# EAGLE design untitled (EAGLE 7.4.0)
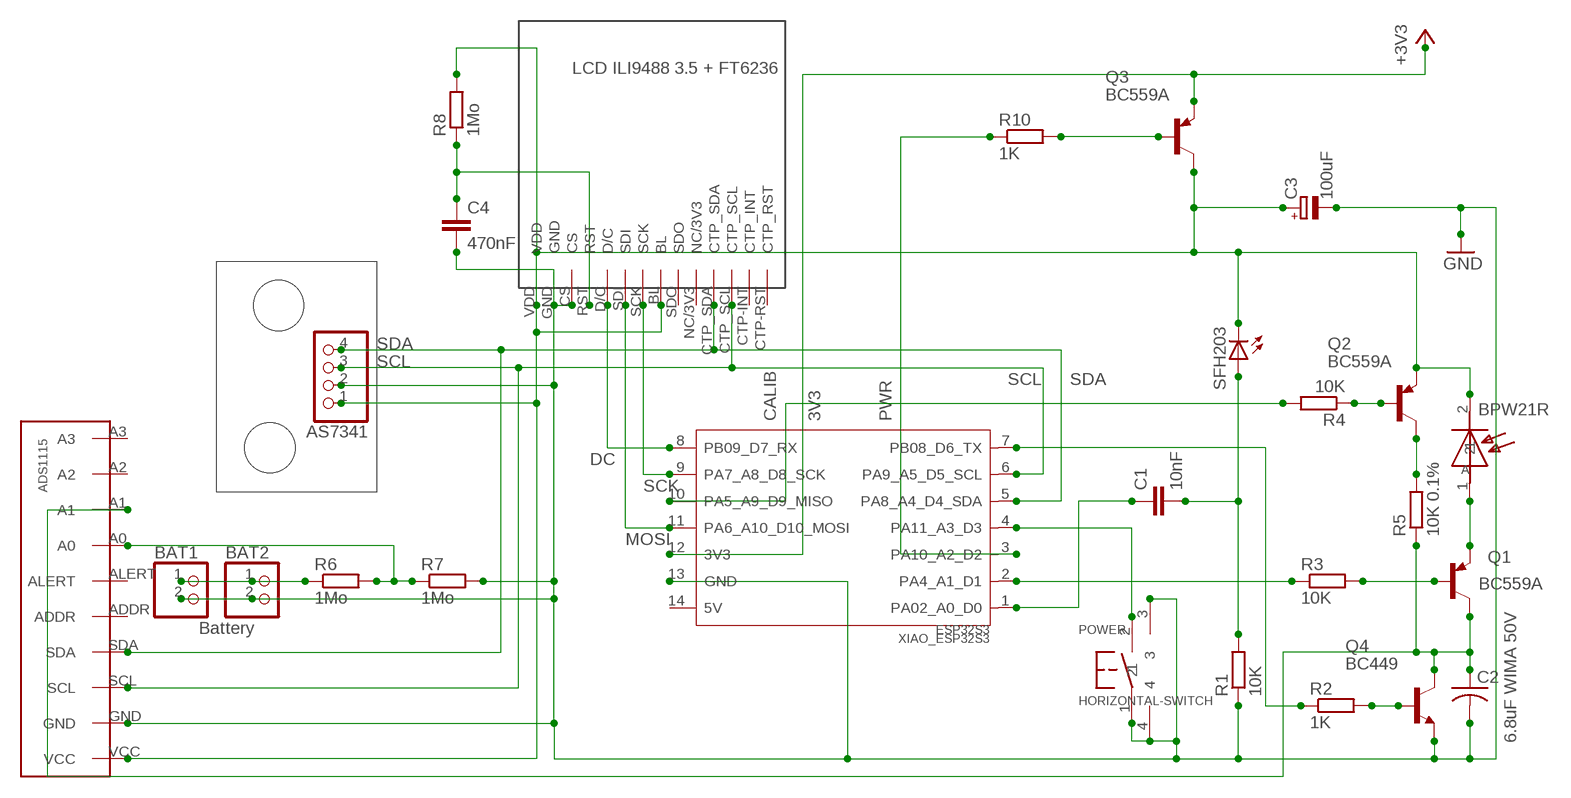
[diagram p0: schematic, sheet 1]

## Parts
ADS1115  HW-ADS1115  [HW-ADS1115]
AS7341  PINHD-1X4  [1X04]
BAT1  PINHD-1X2  [1X02]
BAT2  PINHD-1X2  [1X02]
BPW21R  BPW21  [BPW21]
C1  10nF  C-EU050-025X075  [C050-025X075]
C2  6.8uF WIMA 50V  C-US050-050X075  [C050-050X075]
C3  100uF  CPOL-EUE2.5-6  [E2,5-6]
C4  470nF  C-EU050-025X075  [C050-025X075]
LCD  LCD  IPS-ILI9488-3.5-480-320-FT6236  [IPS-ILI9488-3.5-480-320-FT6236]
POWER  HORIZONTAL-SWITCH  [HORIZONTAL-SWITCH]
Q1  BC559A  [TO92-EBC]
Q2  BC559A  [TO92-EBC]
Q3  BC559A  [TO92-EBC]
Q4  BC449  [TO92-EBC]
R1  10K  R-EU_0207/2V  [0207/2V]
R2  1K  R-EU_0207/2V  [0207/2V]
R3  10K  R-EU_0207/2V  [0207/2V]
R4  10K  R-EU_0207/2V  [0207/2V]
R5  10K 0.1%  R-EU_0207/2V  [0207/2V]
R6  1Mo  R-EU_0207/2V  [0207/2V]
R7  1Mo  R-EU_0207/2V  [0207/2V]
R8  1Mo  R-EU_0207/2V  [0207/2V]
R10  1K  R-EU_0207/2V  [0207/2V]
SFH203  SFH203  [SFH203]
XIAO_ESP32S3  ESP32S3  [MOUDLE14P-2.54-21X17.8MM]

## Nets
+3V3: Q3.E XIAO_ESP32S3.12(3V3)
GND: ADS1115.GND AS7341.2 BAT1.2 BAT2.2 C2.2 C3.- C4.2 LCD.CS LCD.GND POWER.1 POWER.3 POWER.4 Q4.E R1.1 R7.2 XIAO_ESP32S3.13(GND)
N$1: C4.1 LCD.RST R8.1
N$2: C1.1 XIAO_ESP32S3.1(PA02_A0_D0)
N$3: ADS1115.SCL AS7341.3 LCD.CTP_SCL XIAO_ESP32S3.6(PA9_A5_D5_SCL)
N$4: ADS1115.SDA AS7341.4 LCD.CTP_SDA XIAO_ESP32S3.5(PA8_A4_D4_SDA)
N$5: ADS1115.A0 R6.2 R7.1
N$6: LCD.SCK XIAO_ESP32S3.9(PA7_A8_D8_SCK)
N$7: LCD.SDI XIAO_ESP32S3.11(PA6_A10_D10_MOSI)
N$8: LCD.D/C XIAO_ESP32S3.8(PB09_D7_RX)
N$11: R10.1 XIAO_ESP32S3.3(PA10_A2_D2)
N$13: C1.2 R1.2 SFH203.A
N$14: BAT1.1 BAT2.1 R6.1
N$15: Q3.B R10.2
N$17: POWER.2 XIAO_ESP32S3.4(PA11_A3_D3)
N$18: ADS1115.VCC AS7341.1 BPW21R.2 C3.+ LCD.BL LCD.VDD Q2.E Q3.C R8.2 SFH203.K(C)
N$22: Q2.B R4.1
N$23: Q1.B R3.2
N$24: Q4.B R2.2
N$25: ADS1115.A1 C2.1 Q1.C Q4.C R5.1
N$26: Q2.C R5.2
N$27: BPW21R.1 Q1.E
N$29: R4.2 XIAO_ESP32S3.10(PA5_A9_D9_MISO)
N$30: R3.1 XIAO_ESP32S3.2(PA4_A1_D1)
N$31: R2.1 XIAO_ESP32S3.7(PB08_D6_TX)
Unconnected: ADS1115.A2 ADS1115.A3 ADS1115.ADDR ADS1115.ALERT LCD.CTP-INT(CTP_INT) LCD.CTP-RST(CTP_RST) LCD.NC/3V3 LCD.SDO XIAO_ESP32S3.14(5V)

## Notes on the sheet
- LCD ILI9488 3.5 + FT6236
- SDA
- SCL
- SCL | SDA
- CALIB | 3V3 | PWR
- DC
- SCK
- MOSI
- Battery

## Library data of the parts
ADS1115 = perso:HW-ADS1115
AS7341 = pinhead:PINHD-1X4: PIN HEADER
BAT1 BAT2 = pinhead:PINHD-1X2: PIN HEADER
BPW21R = perso:BPW21
C1 C4 = resistor:C-EU: CAPACITOR, European symbol
C2 = resistor:C-US: CAPACITOR, American symbol
C3 = resistor:CPOL-EU: POLARIZED CAPACITOR, European symbol
LCD = perso:IPS-ILI9488-3.5-480-320-FT6236
POWER = perso:HORIZONTAL-SWITCH
Q1-Q3 = transistor-pnp:BC559*: PNP Transistror
Q4 = transistor-npn:BC449*: NPN Transistor
R1-R8 R10 = resistor:R-EU_: RESISTOR, European symbol
SFH203 = perso:SFH203
XIAO_ESP32S3 = Seeed-Studio-XIAO-ESP32S3-footprint-eagle:ESP32S3

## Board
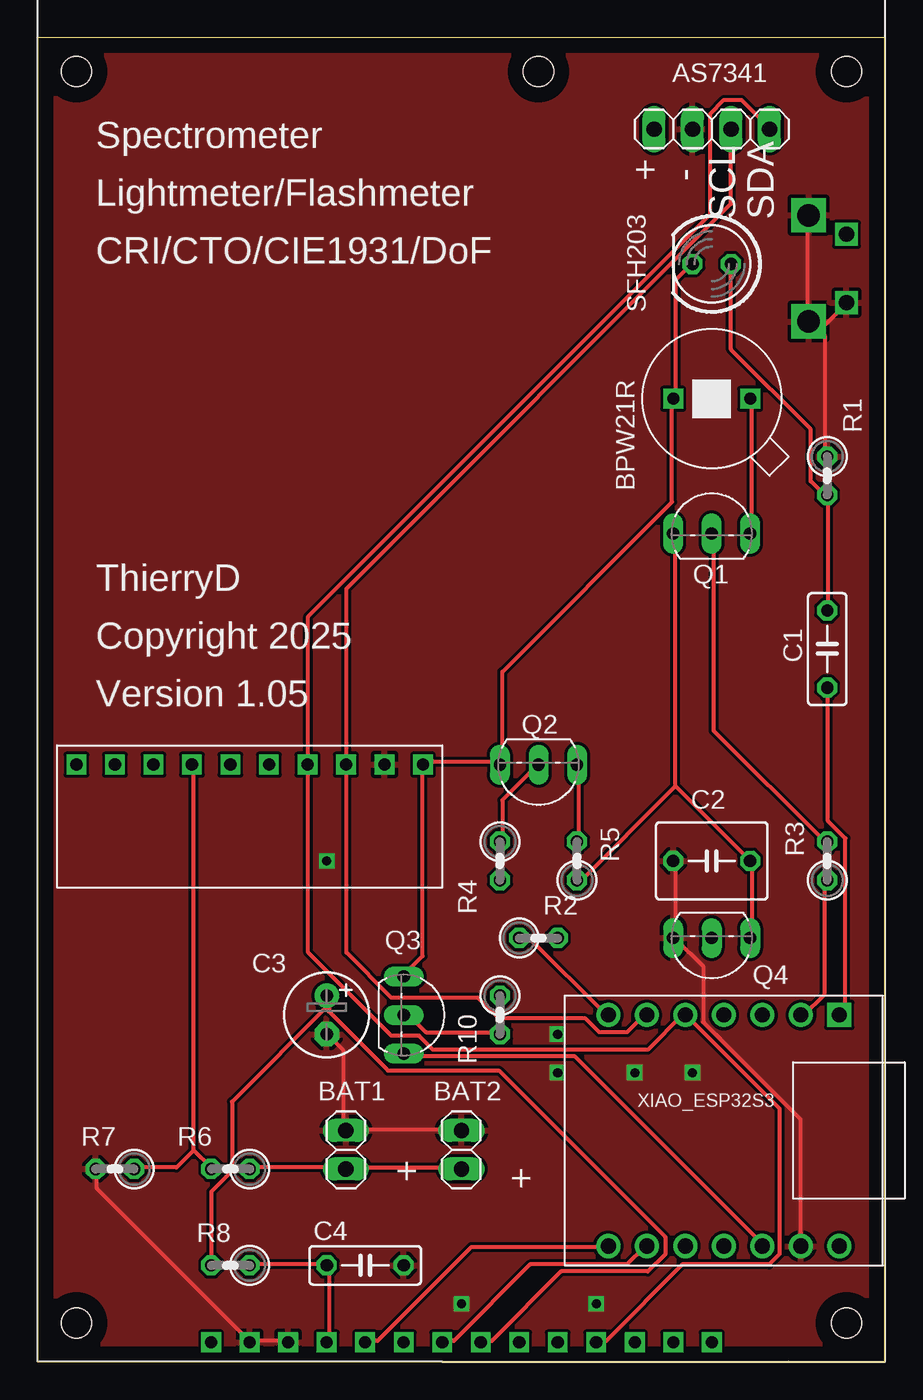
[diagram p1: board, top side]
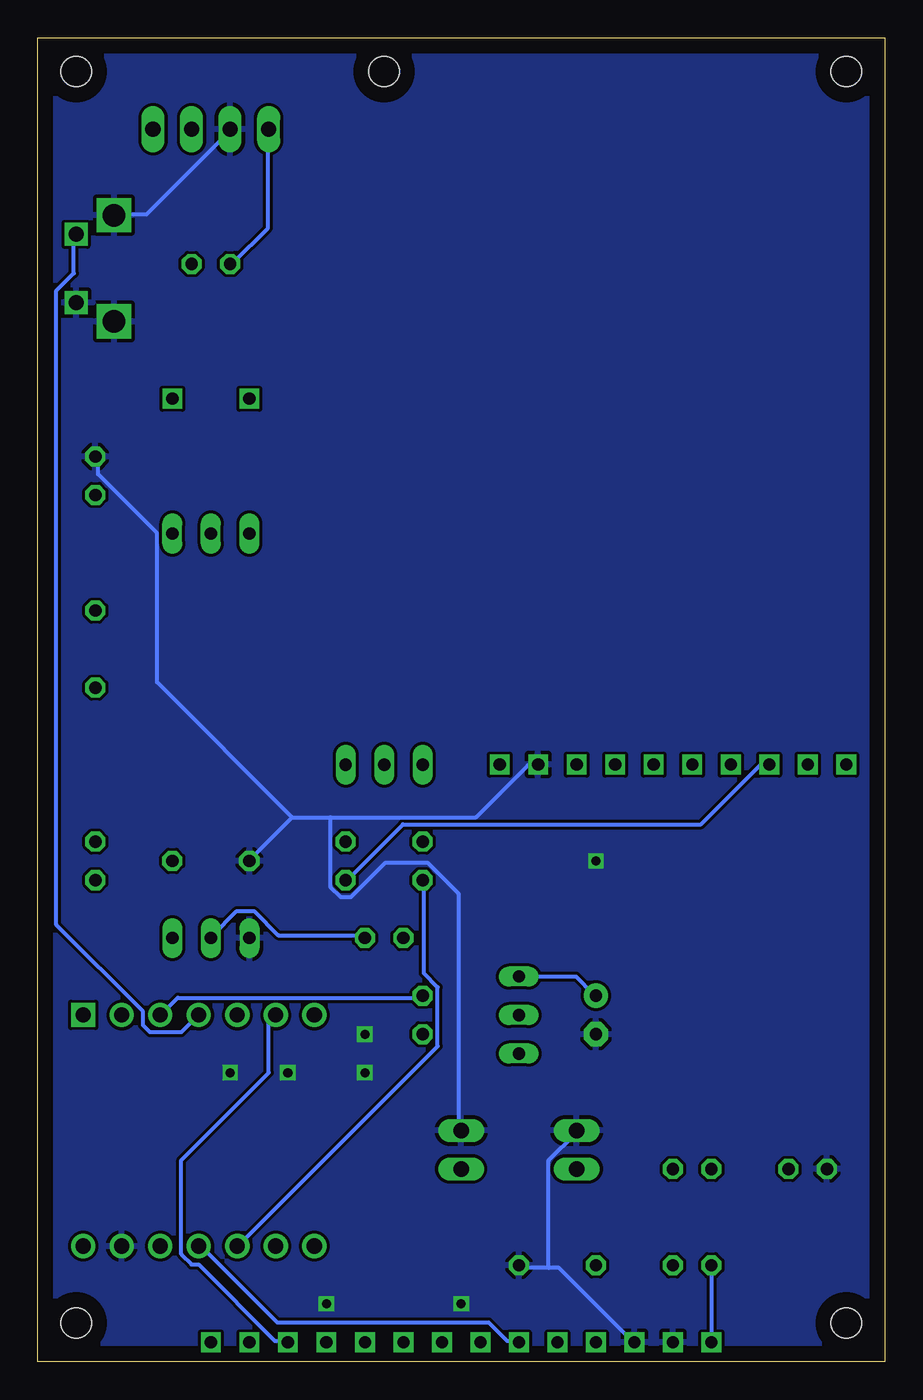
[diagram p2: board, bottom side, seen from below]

Size 55.86 x 87.3 mm. Coordinates in mm from the lower left corner, seen from the top.
Outline: 0,0 55.86,0 55.86,87.3 0,87.3 0,0
Copper layers (1*16): Top 0.035mm / dielectric 1.5mm / Bottom 0.035mm
Design rules "default": minimum track width 10mil, minimum drill 24mil, track to track 8mil, track to pad 8mil, pad to pad 8mil, via to via 8mil, smd to smd 8mil, copper to edge 40mil, drill to drill 8mil, minimum pad ring 10mil, minimum via ring 8mil, stop-mask expansion 4mil, vias tented up to drill 0mil, thermal gap 10mil
Holes 2 mm at 2.54,2.54 53.34,2.54 53.34,85.09 2.54,85.09 33.02,85.09

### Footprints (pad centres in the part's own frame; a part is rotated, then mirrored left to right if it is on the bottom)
HW-ADS1115 = drill 0.8 square: A0 -3.81,0; A1 -6.35,0; A2 -8.89,0; A3 -11.43,0; ADDR 1.27,0; ALERT -1.27,0; GND 8.89,0; SCL 6.35,0; SDA 3.81,0; VCC 11.43,0
1X04 = drill 1.016 long: 1 -3.81,0; 2 -1.27,0; 3 1.27,0; 4 3.81,0
1X02 = drill 1.016 long: 1 -1.27,0; 2 1.27,0
BPW21 = drill 0.8 square: 1 -2.54,0; 2 2.54,0
C050-025X075 = drill 0.813 octagon: 1 -2.54,0; 2 2.54,0
C050-050X075 = drill 0.813 octagon: 1 -2.54,0; 2 2.54,0
E2,5-6 = drill 0.813 pad 1.6: + -1.27,0 | drill 0.813 pad 1.6 octagon: - 1.27,0
IPS-ILI9488-3.5-480-320-FT6236 = drill 0.8 square: BL 1.27,-46.99; CS -11.43,-46.99; CTP-INT 13.97,-46.99; CTP-RST 16.51,-46.99; CTP_SCL 11.43,-46.99; CTP_SDA 8.89,-46.99; D/C -6.35,-46.99; GND -13.97,-46.99; NC/3V3 6.35,-46.99; RST -8.89,-46.99; SCK -1.27,-46.99; SDI -3.81,-46.99; SDO 3.81,-46.99; VDD -16.51,-46.99
HORIZONTAL-SWITCH = drill 1 square: 1 0,0; 2 4.5,0 | drill 1.5 square: 3 -1.25,2.5; 4 5.75,2.5
TO92-EBC = drill 0.813 long: B 0,-1.27; C -2.54,-1.27; E 2.54,-1.27
0207/2V = drill 0.813 octagon: 1 -1.27,0; 2 1.27,0
SFH203 = drill 0.813 octagon: A -1.27,0; K 1.27,0
MOUDLE14P-2.54-21X17.8MM = drill 1 pad 1.6 square: 1 7.62,7.62 | drill 1 pad 1.6: 2 5.08,7.62; 3 2.54,7.62; 4 0,7.62; 5 -2.54,7.62; 6 -5.08,7.62; 7 -7.62,7.62; 8 -7.62,-7.62; 9 -5.08,-7.62; 10 -2.54,-7.62; 11 0,-7.62; 12 2.54,-7.62; 13 5.08,-7.62; 14 7.62,-7.62

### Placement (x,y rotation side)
ADS1115  13.97,39.37 0 top
AS7341  44.45,81.28 0 top
BAT1  20.32,13.97 90 top
BAT2  27.94,13.97 90 top
BPW21R  44.45,63.5 180 top
C1  52.07,46.99 90 top
C2  44.45,33.02 180 top
C3  19.05,22.86 270 top
C4  21.59,6.35 0 top
LCD  27.94,48.26 0 top
POWER  53.34,69.85 90 top
Q1  44.45,55.88 0 top
Q2  33.02,38.1 180 top
Q3  25.4,22.86 270 top
Q4  44.45,26.67 180 top
R1  52.07,58.42 270 top
R2  33.02,27.94 0 top
R3  52.07,33.02 90 top
R4  30.48,33.02 270 top
R5  35.56,33.02 90 top
R6  12.7,12.7 180 top
R7  5.08,12.7 180 top
R8  12.7,6.35 180 top
R10  30.48,22.86 270 top
SFH203  44.45,72.39 180 top
XIAO_ESP32S3  45.25,15.24 0 top

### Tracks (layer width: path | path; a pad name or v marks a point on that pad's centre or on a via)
+3V3
  Top 0.254: Q3.E 24.23,20.12 35.43,20.12 47.78,7.77 XIAO_ESP32S3.12
GND  (via drill 0.6)
  Top 0.254: C3.- 19.2,21.49 20.12,20.57 20.12,15.32 BAT1.2 20.34,15.32 27.89,15.32 BAT2.2 | LCD.CS 16.46,1.37 14.17,1.37 LCD.GND 13.95,1.37 3.89,11.43 3.89,12.57 R7.2 | 51.44,68.12 50.98,68.58 POWER.3 | 51.44,68.12 51.89,67.67 51.89,59.89 R1.1 | 51.44,68.12 51.66,68.12 53.26,69.72 POWER.1 | 51.44,68.12 POWER.3 | POWER.3 50.75,68.81 50.75,75.44 POWER.4 | C2.2 42.06,32.92 42.06,28.12 Q4.E 42.06,27.89 43.89,26.06 43.89,22.4 50.29,16 50.29,7.77 XIAO_ESP32S3.13
  Bottom 0.254: 22.17,6.17 21.49,6.17 16.69,1.37 LCD.CS | 22.17,6.17 24,6.17 C4.2 | 22.17,6.17 22.17,13.26 20.34,15.09 BAT1.2 | AS7341.2 43.2,81.15 48.69,75.67 50.75,75.67 POWER.4 | 39.09,35.89 36.58,35.89 | 36.58,35.89 26.98,35.89 23.55,39.32 22.86,39.32 ADS1115.GND | 39.09,35.89 41.83,33.15 C2.2 | 39.09,35.89 48.01,44.81 48.01,54.63 51.89,58.52 51.89,59.66 R1.1 | 36.58,35.89 36.58,31.32 35.89,30.63 35.2,30.63 32.92,32.92 30.18,32.92 28.12,30.86 28.12,15.32 BAT2.2
  other vias: 19.05,33.02 27.94,3.81 36.83,3.81 43.18,19.05 39.37,19.05 34.29,19.05 34.29,21.59
  pour Top: 0,87.63 55.88,87.63 55.88,0 0,0
  pour Bottom: 0,87.63 55.88,87.63 55.88,0 0,0
N$1
  Top 0.254: LCD.RST 19.2,1.37 19.2,6.17 C4.1 18.97,6.4 14.17,6.4 R8.1
N$2
  Top 0.254: C1.1 52.12,44.35 52.12,35.66 53.26,34.52 53.26,23.09 53.03,22.86 XIAO_ESP32S3.1
N$3
  Top 0.254: XIAO_ESP32S3.6 40.01,22.86 38.86,21.72 37.03,21.72 36.12,22.63 30.4,22.63 29.03,24 23.32,24 20.34,26.98 20.34,39.32 ADS1115.SCL 20.34,39.55 20.34,50.98 45.72,76.35 AS7341.3
  Bottom 0.254: LCD.CTP_SCL 39.55,1.37 40.23,1.37 45.26,6.4 45.72,6.4 46.41,7.09 46.41,13.28 40.64,19.05 40.64,22.39 XIAO_ESP32S3.6 40.23,22.86
N$4
  Top 0.254: LCD.CTP_SDA 37.03,1.37 37.49,1.37 42.52,6.4 48.23,6.4 48.92,7.09 48.92,16.69 42.75,22.86 XIAO_ESP32S3.5 42.52,22.86 40.23,20.57 26.06,20.57 25.15,21.49 23.32,21.49 17.83,26.98 17.83,39.32 ADS1115.SDA 17.83,39.55 17.83,49.15 44.35,75.67 44.35,82.3 45.26,83.21 46.41,83.21 48.23,81.38 AS7341.4
N$5
  Top 0.254: 10.29,13.95 10.29,39.32 ADS1115.A0 | 10.29,13.95 11.43,12.8 R6.2 | 10.29,13.95 9.14,12.8 6.4,12.8 R7.1
N$6
  Top 0.254: LCD.SCK 26.75,1.37 27.43,1.37 32.46,6.4 38.86,6.4 40.01,7.54 XIAO_ESP32S3.9
N$7
  Bottom 0.254: LCD.SDI 24.23,1.37 24.92,1.37 26.14,2.59 40.08,2.59 45.03,7.54 XIAO_ESP32S3.11
N$8
  Top 0.254: LCD.D/C 21.72,1.37 22.4,1.37 28.57,7.54 37.49,7.54 XIAO_ESP32S3.8
N$11
  Bottom 0.254: R10.1 30.63,24 46.63,24 47.78,22.86 XIAO_ESP32S3.3
N$13
  Top 0.254: C1.2 52.12,49.61 52.12,57.15 R1.2 51.89,57.15 50.98,58.06 50.98,61.49 45.72,66.75 SFH203.A
N$14
  Top 0.254: R6.1 14.17,12.8 20.12,12.8 BAT1.1 20.34,12.8 27.89,12.8 BAT2.1
N$15
  Top 0.254: Q3.B 24.46,22.86 25.6,21.72 30.4,21.72 R10.2
N$17
  Bottom 0.254: POWER.2 53.49,74.3 53.49,71.78 54.63,70.64 54.63,28.8 48.92,23.09 48.92,22.17 48.46,21.72 46.41,21.72 45.26,22.86 XIAO_ESP32S3.4
N$18
  Top 0.254: SFH203.K 42.98,72.24 42.06,71.32 42.06,63.55 BPW21R.2 41.83,63.32 41.83,56.69 30.63,45.49 30.63,39.55 Q2.E 30.4,39.55 25.6,39.55 ADS1115.VCC 25.38,39.32 25.38,26.75 24.23,25.6 Q3.C | 19.2,23.55 19.2,24 C3.+ 19.2,23.55 | 19.2,23.55 19.2,23.09 23.09,19.2 30.4,19.2 41.38,8.23 41.38,7.09 40.23,5.94 34.52,5.94 29.95,1.37 29.26,1.37 LCD.BL | R8.2 11.43,11.2 12.8,12.57 12.8,17.14 19.2,23.55
  Bottom 0.254: AS7341.1 40.69,81.15 40.69,74.75 42.98,72.47 SFH203.K | R8.2 LCD.VDD | Q3.C 24,25.38 20.34,25.38 19.2,24.23 C3.+
N$22
  Top 0.254: R4.1 30.63,34.29 30.63,37.03 32.92,39.32 Q2.B
N$23
  Top 0.254: Q1.B 44.58,54.41 44.58,41.6 51.89,34.29 R3.2
N$24
  Bottom 0.254: R2.2 34.29,28.12 40.01,28.12 41.6,29.72 42.75,29.72 44.35,28.12 Q4.B
N$25
  Top 0.254: Q4.C 47.09,28.12 47.09,32.92 C2.1 42.06,37.95 | 42.06,37.95 42.06,54.41 Q1.C | 42.06,37.95 35.66,31.55 R5.1
  Bottom 0.254: ADS1115.A1 7.77,39.32 8.23,39.32 12.12,35.43 31.77,35.43 35.43,31.77 R5.1
N$26
  Top 0.254: R5.2 35.66,34.29 35.66,39.32 Q2.C
N$27
  Top 0.254: BPW21R.1 47.09,63.32 47.09,54.63 Q1.E
N$29
  Bottom 0.254: R4.2 30.4,31.55 30.4,25.6 29.49,24.69 29.49,20.8 42.52,7.77 XIAO_ESP32S3.10
N$30
  Top 0.254: R3.1 51.89,31.55 51.89,24.23 50.52,22.86 XIAO_ESP32S3.2
N$31
  Top 0.254: R2.1 31.77,27.89 32.46,27.89 37.49,22.86 XIAO_ESP32S3.7

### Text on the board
tNames: Spectrometer | + | - | Lightmeter/Flashmeter | SCL | SDA | CRI/CTO/CIE1931/DoF | ThierryD | Copyright 2025 | Version 1.05 | + | +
